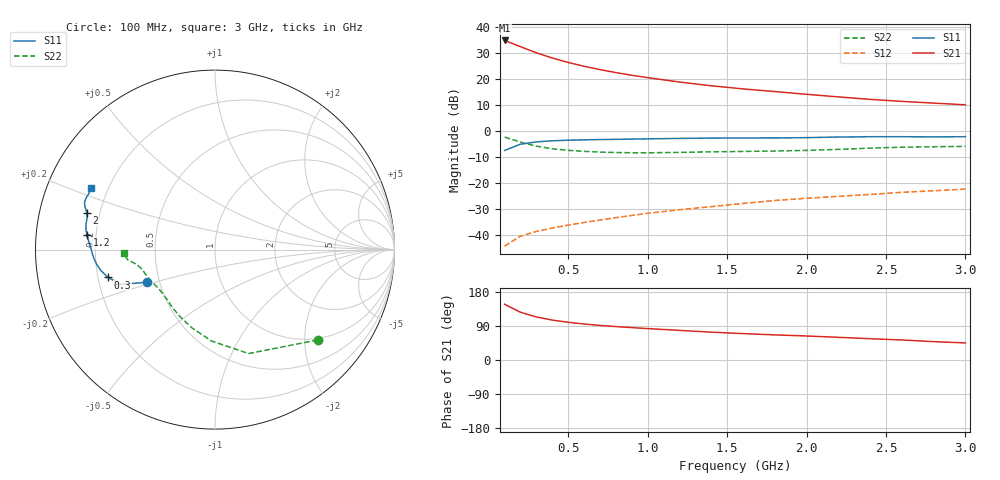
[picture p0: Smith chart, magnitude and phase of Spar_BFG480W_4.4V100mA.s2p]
! Filename: 4_4100BFG480.001
! Title: BFG480W
! Bias: Vce=4.4V; Ic=100mA
! Company: NXP Semiconductors NL
! User: Quality&Reliability T&D
! Measure time: 10 Nov 1999 / 12:07:04
#  MHz  S  MA  R 50
! Freq  S11  S21  S12  S22  :
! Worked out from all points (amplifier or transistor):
!   20 points, 100 MHz to 3 GHz, reference 50 ohm
!   highest |S21| = 34.7 dB at 100 MHz (marker M1)
!   |S21| within 3 dB of that: start of sweep to 226.5 MHz
!   unconditionally stable (mu >= 1): 725.3 MHz to end of sweep
!   at 400 MHz: K = 0.80, MSG = 32.6 dB, |S12| = -37.2 dB
!   at 1.2 GHz: K = 1.07, MAG = 22.8 dB, |S12| = -30.2 dB
!   at 3 GHz: K = 1.04, MAG = 14.9 dB, |S12| = -22.3 dB
!   S11 on the Smith chart (normalised r, x): 100 MHz: 0.42, -0.19; 300 MHz: 0.24, -0.12; 1.2 GHz: 0.16, +0.06; 2 GHz: 0.15, +0.14; 3 GHz: 0.13, +0.23
100  0.4225 -154.5  54.19 147.2  0.006175 68.5  0.7616 -41.4
200  0.5563 -159.6  41.2 125.9  0.009615 60.6  0.6086 -72.1
300  0.6163 -165.4  31.45 113.5  0.01183 59.2  0.5094 -92.3
400  0.6463 -169.6  24.96 105.4  0.01374 60.8  0.4548 -106.3
500  0.6638 -172.8  20.54 99.5  0.01565 62.7  0.424 -116.5
600  0.675 -175.5  17.33 95.0  0.01755 64.7  0.4053 -124.0
700  0.6827 -177.8  14.97 91.3  0.01955 66.9  0.393 -130.0
800  0.6894 -179.9  13.13 88.2  0.02175 68.8  0.3851 -134.9
900  0.6963 178.2  11.67 85.5  0.02395 70.7  0.3812 -139.2
1000  0.7046 176.4  10.49 82.9  0.0263 71.6  0.3805 -143.0
1200  0.7179 173.4  8.656 78.2  0.03084 73.3  0.3873 -149.2
1400  0.728 171.1  7.329 73.5  0.03536 74.3  0.3976 -153.8
1600  0.7329 168.7  6.392 69.7  0.04063 75.1  0.404 -157.3
1800  0.7338 166.1  5.681 66.3  0.04631 75.7  0.4116 -161.0
2000  0.7433 163.9  5.029 63.3  0.05116 76.4  0.423 -165.4
2200  0.7625 161.8  4.489 59.9  0.05558 76.3  0.4427 -169.1
2400  0.7737 160.0  4.025 56.2  0.06047 75.8  0.4676 -171.5
2600  0.7738 158.4  3.68 52.8  0.06656 75.2  0.4871 -173.0
2800  0.7691 156.1  3.412 48.5  0.07131 73.8  0.497 -174.8
3000  0.7741 153.5  3.17 45.1  0.07674 73.0  0.5048 -177.6
